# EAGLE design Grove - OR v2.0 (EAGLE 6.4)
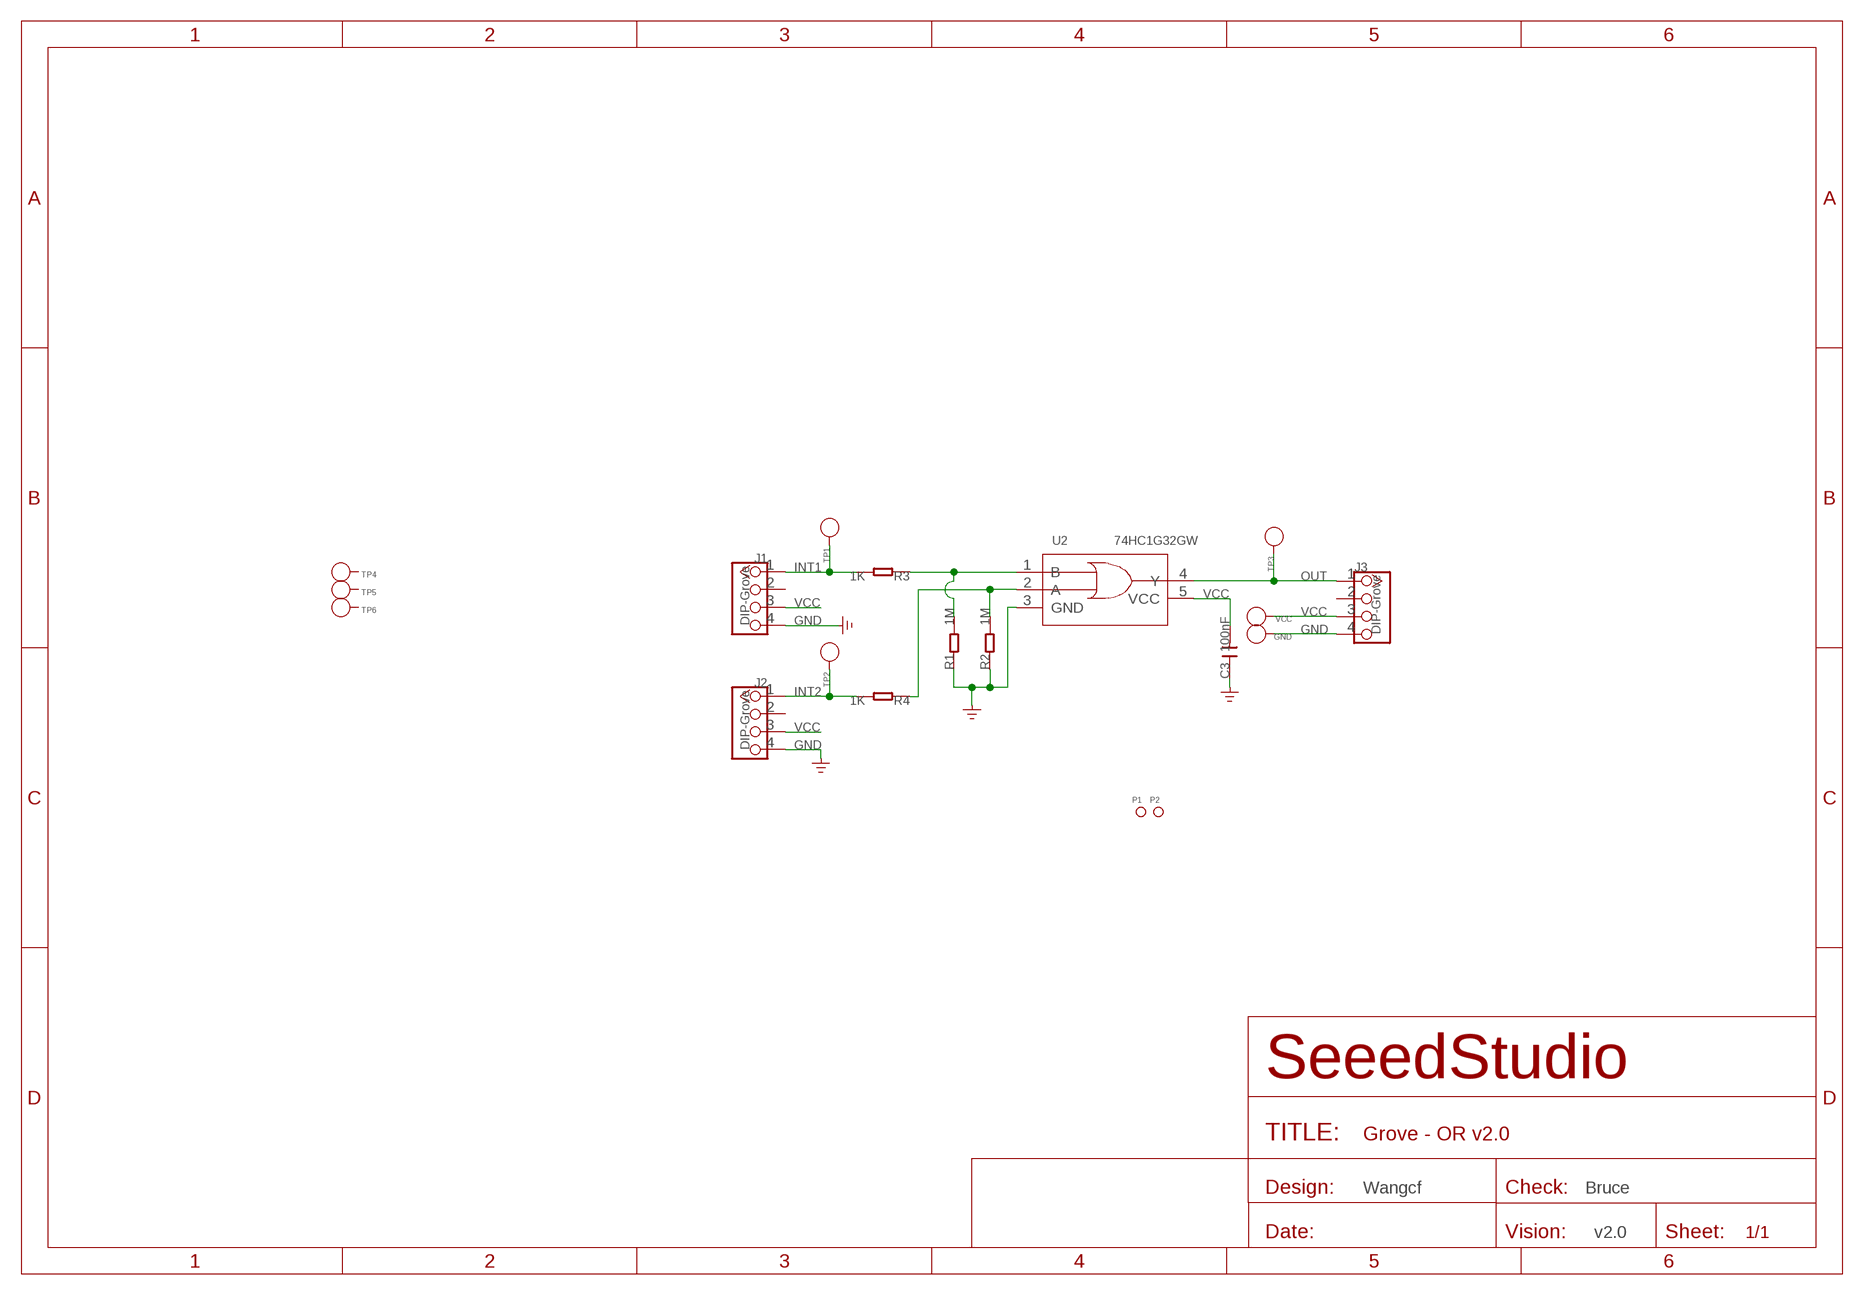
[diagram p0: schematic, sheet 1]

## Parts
C3  100nF  C-0603  [C0603]
GND  PAD-TEST-POINT'4545'  [TP_4545]
J1  DIP-Grove  TWIG-4P-2.0-2.0  [4P-2.0]
J2  DIP-Grove  TWIG-4P-2.0-2.0  [4P-2.0]
J3  DIP-Grove  TWIG-4P-2.0-2.0  [4P-2.0]
P1  PAD-MARK  [ROUND-MARK-1.0]
P2  PAD-MARK  [ROUND-MARK-1.0]
R1  1M  R-0603  [R0603]
R2  1M  R-0603  [R0603]
R3  1K  R-0603  [R0603]
R4  1K  R-0603  [R0603]
TP1  PAD-TEST-POINT'4545'  [TP_4545]
TP2  PAD-TEST-POINT'4545'  [TP_4545]
TP3  PAD-TEST-POINT'4545'  [TP_4545]
TP4  PAD-TEST-POINT'4545'  [TP_4545]
TP5  PAD-TEST-POINT'4545'  [TP_4545]
TP6  PAD-TEST-POINT'4545'  [TP_4545]
U2  74HC1G32GW  74HC1G32'GW'  [SOT-353]
VCC  PAD-TEST-POINT'4545'  [TP_4545]

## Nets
GND: C3.1 GND.T J1.4 J2.4 J3.4 R1.1 R2.1 U2.3(GND)
INT1: J1.1 R3.2 TP1.T
INT2: J2.1 R4.2 TP2.T
N$4: R2.2 R4.1 U2.2(A)
N$21: R1.2 R3.1 U2.1(B)
OUT: J3.1 TP3.T U2.4(Y)
VCC: C3.2 J1.3 J2.3 J3.3 U2.5(VCC) VCC.T
Unconnected: J1.2 J2.2 J3.2 TP4.T TP5.T TP6.T

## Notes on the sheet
- Wangcf | Bruce
- v2.0

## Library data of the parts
C3 = Discrete:C*: Ceramic Capacitors
GND TP1-TP6 VCC = Discrete:PAD-TEST-POINT; PARTNO: DNP
J1-J3 = Connector :TWIG-4P-2.0
P1 P2 = Discrete:PAD-MARK; PARTNO: DNP
R1-R4 = Discrete:R*
U2 = template:74HC1G32: 2-input OR gate

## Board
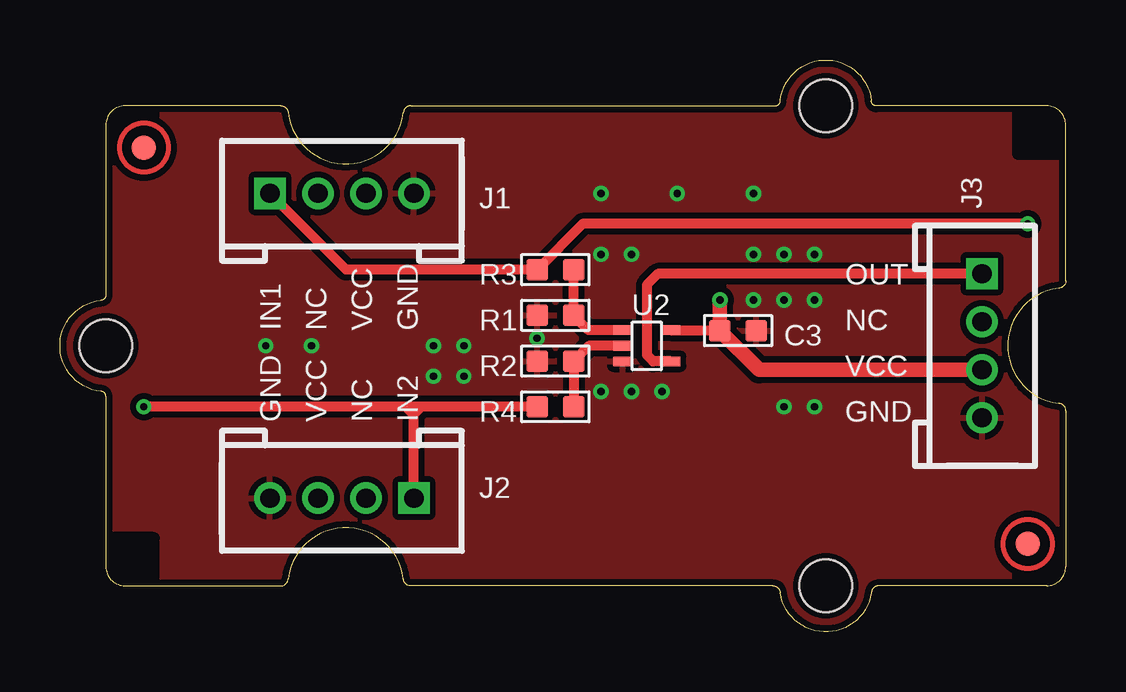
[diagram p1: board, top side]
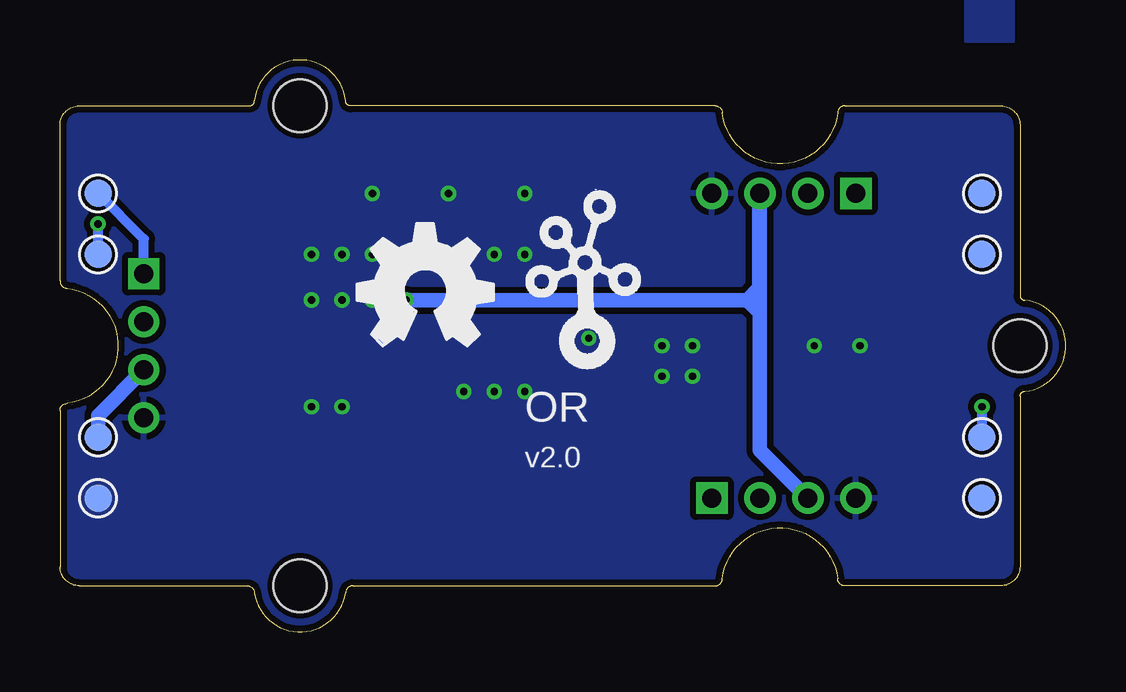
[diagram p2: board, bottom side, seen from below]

Size 41.91 x 23.83 mm. Coordinates in mm from the lower left corner, seen from the top.
Copper layers (1*16): Top 0.035mm / dielectric 1.5mm / Bottom 0.035mm
Design rules "SeeedStudio_DRU_no_angle_20130527 *": minimum track width 6mil, minimum drill 12mil, track to track 6mil, track to pad 6mil, pad to pad 6mil, via to via 6mil, smd to smd 0mil, copper to edge 10mil, drill to drill 10mil, minimum pad ring 10mil, minimum via ring 6mil, stop-mask expansion 2mil, vias tented up to drill 25mil, thermal gap 10mil

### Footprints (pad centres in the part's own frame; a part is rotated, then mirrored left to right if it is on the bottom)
C0603 = smd 0.889 x 0.889: 1 -0.762,0; 2 0.762,0
TP_4545 = smd 1.143 x 1.143: T 0,0
4P-2.0 = drill 0.8 pad 1.27 square: 1 -3,0 | drill 0.8 pad 1.27: 2 -1,0; 3 1,0; 4 3,0
ROUND-MARK-1.0 = smd 1.016 x 1.016: P$1 0,0
R0603 = smd 0.889 x 0.889: 1 -0.762,0; 2 0.762,0
SOT-353 = smd 0.4 x 0.8: 1 -0.65,-1; 2 0,-1; 3 0.65,-1; 4 0.65,1; 5 -0.65,1
GROVE-3CONNECTOR-FIRST = hole 2.2: -10,-10; -10,10; 20,0

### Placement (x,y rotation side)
C3  28.26,12.56 180 top
GND  40.32,5.57 0 bottom
J1  11.75,18.27 0 top
J2  11.75,5.57 180 top
J3  38.42,11.92 270 top
P1  3.49,20.18 0 top
P2  40.32,3.67 0 top
R1  20.64,13.19 0 top
R2  20.64,11.29 0 top
R3  20.64,15.1 180 top
R4  20.64,9.38 180 top
TP1  40.32,15.73 0 bottom
TP2  3.49,8.11 0 bottom
TP3  40.32,18.27 0 bottom
TP4  3.49,18.27 0 bottom
TP5  3.49,15.73 0 bottom
TP6  3.49,5.57 0 bottom
U2  24.45,11.92 270 top
U$2  [GROVE-3CONNECTOR-FIRST]  21.91,11.92 180 top
U$3  [OSHW_FILLX200_NOTEXT]  29.53,11.92 0 bottom
U$4  [TWIGLOGO]  20,11.92 0 bottom
VCC  40.32,8.11 0 bottom

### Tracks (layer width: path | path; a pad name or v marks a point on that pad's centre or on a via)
GND  (via drill 0.3 pad 0.64)
  other vias: 28.89,13.83 30.16,13.83 31.43,13.83 22.54,10.02 23.81,10.02 25.08,10.02 28.89,15.73 30.16,15.73 31.43,15.73 16.83,11.92 16.83,10.65 15.56,10.65 15.56,11.92 10.48,11.92 8.57,11.92 19.88,12.24 22.54,15.73 23.81,15.73 22.54,18.27 28.89,18.27 25.72,18.27 31.43,9.38 30.16,9.38
  pour Bottom: 2.22,24.62 4.13,24.62 4.13,26.53 2.22,26.53
  pour Top (isolate 0.254): -0.32,23.35 -0.32,23.99 42.23,23.99 42.23,-0.14 -0.32,-0.14
  pour Bottom (isolate 0.254): -0.32,23.35 -0.32,23.99 42.23,23.99 42.23,-0.14 -0.32,-0.14
INT1  (via drill 0.3 pad 0.64)
  Top 0.406: v40.32,17 21.78,17 R3.2 11.92,15.1 J1.1
  Bottom 0.406: TP1.T v40.32,17
INT2  (via drill 0.3 pad 0.64)
  Top 0.406: R4.2 15.05,9.38 | 14.67,9.38 14.42,9.38 | 14.42,9.38 v3.49,9.38 | J2.1 14.75,9.05 | 14.75,9.08 14.75,9.3 14.67,9.38 | 14.75,9.05 14.42,9.38 | 14.75,9.05 14.75,9.08 | 14.75,9.08 15.05,9.38 | 15.05,9.38 14.67,9.38
  Bottom 0.406: v3.49,9.38 TP2.T
N$4
  Top 0.406: U2.2 22.04,11.92 R2.2 R4.1
N$21
  Top 0.406: U2.1 22.02,12.57 R1.2 R3.1
OUT
  Top 0.406: J3.1 24.91,14.92 24.45,14.46 24.45,11.54 24.72,11.27 U2.4
  Bottom 0.406: J3.1 38.42,16.37 TP3.T
VCC  (via drill 0.3 pad 0.64)
  Top 0.406: U2.5 27.48,12.57 C3.2
  Top 0.61: J3.3 29.13,10.92 C3.2 v27.5,13.83
  Bottom 0.61: v27.5,13.83 13.27,13.83 | 13.27,13.83 12.76,13.83 | J2.3 12.75,7.57 J1.3 12.76,18.26 12.76,14.33 | 12.76,13.83 12.76,14.33 | VCC.T 40.32,9.02 J3.3 | 13.27,13.83 12.76,14.33 | 13.27,13.83 12.76,13.32 12.76,13.83

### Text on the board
tPlace: OUT | IN1 | NC | VCC | GND | NC | VCC | GND | VCC | NC | IN2 | GND
bPlace: OR | v2.0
